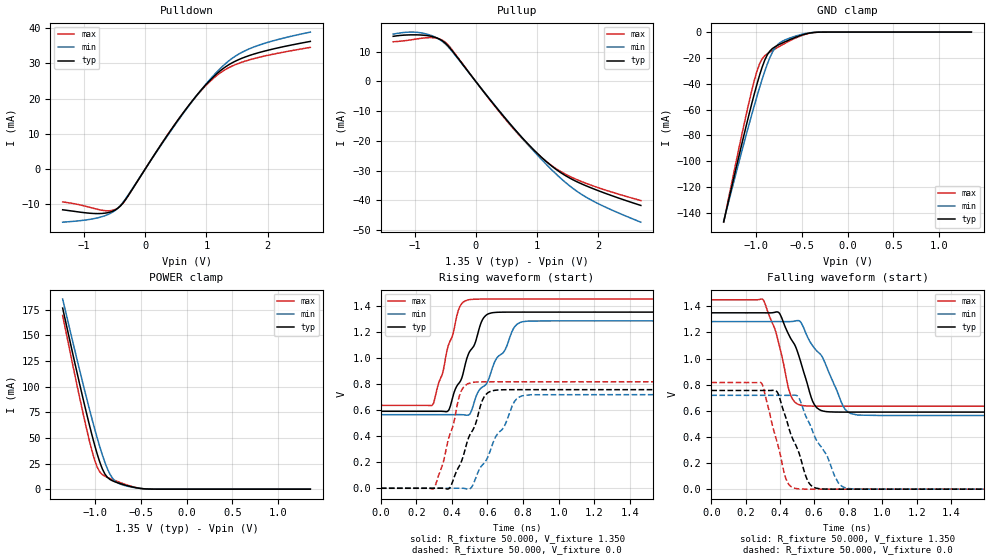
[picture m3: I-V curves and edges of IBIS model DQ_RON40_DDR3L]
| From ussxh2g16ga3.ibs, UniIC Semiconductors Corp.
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|   Model DQ_RON40_DDR3L
[Model] DQ_RON40_DDR3L
Model_type I/O
Vinl =  0.540V
Vinh =  0.810V
Vmeas =  0.675V
Rref =  50.000
Vref =  0.675V
C_comp   0.966pF   0.965pF   0.967pF
[Model Spec]
Vinh   0.810V   0.776V   0.860V
Vinl   0.540V   0.506V   0.590V
Vmeas   0.675V   0.641V   0.725V
Vref   0.675V   0.641V   0.725V
Rref   50.000   NA   NA
[Temperature Range]   25.000   95.000   -40.000
[Voltage Range]   1.350V   1.283V   1.450V
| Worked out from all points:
|   slope of the pulldown table from 0 to 0.203 V, typ, clamps not added: 37.2 ohm
|   slope of the pullup table from 0 to 0.203 V, typ, clamps not added: 38 ohm
|   GND clamp passes 1 mA (typ) near -0.43 V on its own axis
|   POWER clamp passes 1 mA (typ) near -0.52 V on its own axis
|   rising waveform, R_fixture 50.000, V_fixture 1.350: 20-80 % time 134ps typ, 184ps min, 98.3ps max; typ from 0.59 V to 1.35 V
|   rising waveform, R_fixture 50.000, V_fixture 0.0: 20-80 % time 121ps typ, 170ps min, 89.2ps max; typ from 0 V to 0.756 V
|   falling waveform, R_fixture 50.000, V_fixture 1.350: 20-80 % time 128ps typ, 175ps min, 95.1ps max; typ from 1.35 V to 0.59 V
|   falling waveform, R_fixture 50.000, V_fixture 0.0: 20-80 % time 119ps typ, 161ps min, 92ps max; typ from 0.756 V to 0 V
[Pulldown]
|Voltage   I(typ)   I(min)   I(max)
-1.35V    -11.58mA   -15.1mA    -9.345mA
-735mV    -12.64mA   -13.67mA   -11.62mA
-571mV    -12.21mA   -12.61mA   -11.84mA
-448mV    -11.14mA   -11.13mA   -11.09mA
-325mV    -8.759mA   -8.551mA   -8.829mA
249mV     6.658mA    6.511mA    6.715mA
618mV     15.87mA    15.68mA    15.89mA
905mV     22.23mA    22.23mA    22.07mA
1.151V    26.74mA    27.18mA    26.28mA
1.397V    29.91mA    31.1mA     29.03mA
1.684V    32.11mA    33.98mA    30.89mA
2.7V      36.23mA    38.87mA    34.53mA
[Pullup]
|Voltage   I(typ)   I(min)   I(max)
-1.35V    15.19mA    15.93mA    13.35mA
-908mV    15.63mA    16.4mA     14.47mA
-703mV    15.07mA    15.27mA    14.72mA
-539mV    13.58mA    13.35mA    13.78mA
-416mV    11.12mA    10.85mA    11.42mA
568mV     -14.48mA   -14.45mA   -14.75mA
855mV     -21.05mA   -21.3mA    -21.28mA
1.142V    -26.78mA   -27.68mA   -26.77mA
1.429V    -31.24mA   -33.33mA   -30.81mA
1.757V    -34.74mA   -38.38mA   -33.95mA
2.126V    -37.73mA   -42.38mA   -36.62mA
2.7V      -41.76mA   -47.4mA    -40.11mA
[GND_clamp]
|Voltage   I(typ)   I(min)   I(max)
-1.35V    -146.9mA   -146.3mA   -147.1mA
-1.126V   -78.8mA    -85.17mA   -70.77mA
-1.014V   -47.25mA   -56.31mA   -36.92mA
-958mV    -33.17mA   -42.77mA   -24.44mA
-930mV    -26.97mA   -36.36mA   -20.61mA
-874mV    -17.51mA   -24.69mA   -16.72mA
-818mV    -12.71mA   -15.46mA   -14.21mA
-762mV    -10.26mA   -9.751mA   -11.88mA
-706mV    -8.307mA   -6.907mA   -9.644mA
-538mV    -3.274mA   -2.499mA   -3.731mA
-398mV    -591.2uA   -439.3uA   -663.7uA
1.35V     0A         0A         0A
[POWER_clamp]
|Voltage   I(typ)   I(min)   I(max)
-1.35V    176.6mA    185.4mA    169.4mA
-1.198V   115.5mA    128.2mA    103.2mA
-1.114V   83.04mA    97.6mA     68.48mA
-1.058V   62.42mA    77.92mA    46.98mA
-1.002V   43.19mA    59.09mA    28.56mA
-946mV    26.54mA    41.57mA    16.92mA
-890mV    14.85mA    26.22mA    12.66mA
-834mV    9.439mA    14.55mA    10.39mA
-778mV    7.089mA    7.901mA    8.361mA
-638mV    3.198mA    2.764mA    3.815mA
-414mV    126.6uA    165.9uA    94.28uA
1.35V     0A         0A         0A
[Ramp]
| variable   typ   min   max
dV/dt_r   0.453/0.121n   0.431/0.169n   0.490/88.918p
dV/dt_f   0.456/0.128n   0.431/0.176n   0.489/95.090p
R_load = 50.000
[Rising Waveform]
R_fixture= 50.000
V_fixture= 1.350
V_fixture_min= 1.283
V_fixture_max= 1.450
|time   V(typ)   V(min)   V(max)
0s        589.8mV    563.9mV    635.3mV
288ps     589.8mV    563.9mV    634.2mV
348ps     589.5mV    563.9mV    883.5mV
380ps     594.4mV    563.8mV    1.095V
441ps     807.9mV    564.2mV    1.381V
494ps     1.033V     561.4mV    1.444V
592ps     1.326V     796.5mV    1.45V
745ps     1.35V      1.221V     1.45V
797ps     1.35V      1.276V     1.45V
3ns       1.35V      1.283V     1.45V
[Rising Waveform]
R_fixture= 50.000
V_fixture= 0.0
V_fixture_min= 0.0
V_fixture_max= 0.0
|time   V(typ)   V(min)   V(max)
0s        148nV      998nV      75.27nV
299ps     -65.85uV   2.446uV    503.1uV
348ps     150.4uV    5.9uV      183.5mV
389ps     5.228mV    -48.25uV   414.7mV
451ps     196.8mV    513uV      740.2mV
511ps     432.5mV    8.863mV    809.9mV
597ps     726.2mV    225.1mV    815.9mV
752ps     755.6mV    665.2mV    816.1mV
795ps     755.6mV    708.3mV    816.1mV
3ns       755.6mV    718.3mV    816.1mV
[Falling Waveform]
R_fixture= 50.000
V_fixture= 1.350
V_fixture_min= 1.283
V_fixture_max= 1.450
|time   V(typ)   V(min)   V(max)
0s        1.35V      1.283V     1.45V
305ps     1.35V      1.283V     1.446V
397ps     1.349V     1.283V     1.102V
463ps     1.156V     1.283V     722mV
524ps     967.5mV    1.276V     642.6mV
616ps     623.8mV    1.059V     635.4mV
654ps     597.7mV    998.6mV    635.3mV
773ps     589.9mV    628.9mV    635.3mV
815ps     589.8mV    578.6mV    635.3mV
3ns       589.8mV    563.9mV    635.3mV
[Falling Waveform]
R_fixture= 50.000
V_fixture= 0.0
V_fixture_min= 0.0
V_fixture_max= 0.0
|time   V(typ)   V(min)   V(max)
0s        755.6mV    718.3mV    816.1mV
292ps     755.6mV    718.3mV    813.9mV
384ps     745.6mV    718.3mV    362.2mV
436ps     545.7mV    718.1mV    79.75mV
491ps     344.6mV    719.6mV    6.183mV
512ps     279.2mV    698.9mV    2.233mV
582ps     29.65mV    478.2mV    76.1uV
741ps     30.01uV    50.75mV    250.7nV
787ps     4.187uV    8.759mV    210.4nV
3ns       95.89nV    981nV      147.6nV
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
